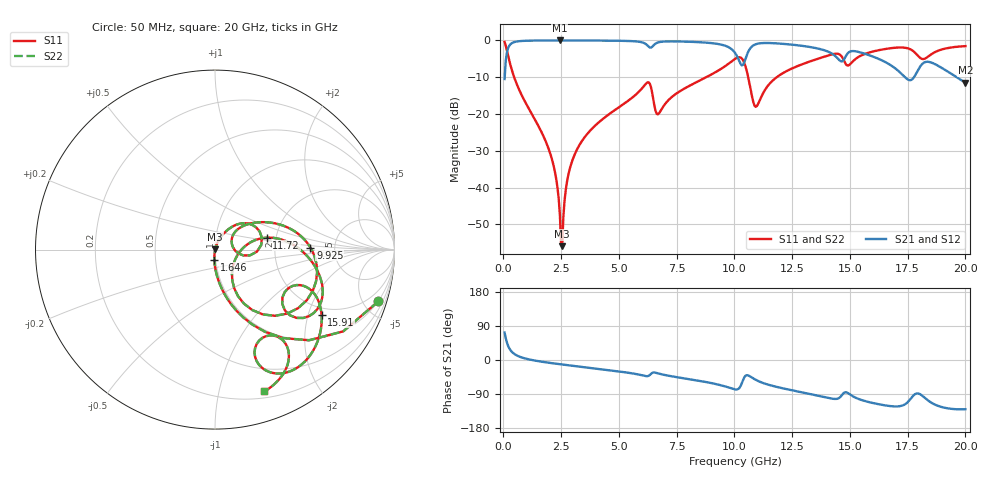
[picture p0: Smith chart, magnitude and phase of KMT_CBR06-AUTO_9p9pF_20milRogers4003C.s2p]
! Data measured by Modelithics Inc. support@modelithics.com 813-866-6335
! KEMET CBR06-AUTO 9.9pF, Pad Width= 0.851mm, Pad Length= 0.64mm, Pad Gap= 0.62mm, 20mil Rogers 4003C substrate Data, January 2022
# hz S ma R 50
! 2 Port Network Data from SP1.SP block
! freq  magS11  angS11  magS21  angS21  magS12  angS12  magS22  angS22
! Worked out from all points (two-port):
!   401 points, 50 MHz to 20 GHz, reference 50 ohm
!   highest |S21| = -0.01 dB at 2.444 GHz (marker M1); lowest = -11.5 dB at 20 GHz (marker M2)
!   |S21| within 3 dB of the highest: 161.7 MHz to 9.978 GHz (9.817 GHz wide, 194 % of centre); 10.6 GHz to 14.04 GHz (3.435 GHz wide, 27.9 % of centre)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
!   lowest |S11| = -55.9 dB at 2.544 GHz (marker M3), VSWR 1.00, Z = 50.1 + j0.102 ohm
!   |S11| at or under -10 dB: 463.8 MHz to 8.779 GHz (8.315 GHz wide, 180 % of centre); 10.6 GHz to 11.83 GHz (1.237 GHz wide, 11 % of centre)
!   |S22| runs from -55.9 to -0.4 dB; largest |S21 - S12| = 0
!   S11 on the Smith chart (normalised r, x): 50 MHz: 0.98, -6.30; 1.646 GHz: 0.99, -0.11; 9.925 GHz: 3.27, +0.10; 11.72 GHz: 1.79, +0.26; 15.91 GHz: 1.75, -2.45; 20 GHz: 0.26, -1.37
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5e7  0.9542 -17.6  0.2989 72.4  0.2989 72.4  0.9542 -17.6
4.49e8  0.3259 -73.0  0.9448 16.9  0.9448 16.9  0.3259 -73.0
1.646e9  0.05689 -93.6  0.9975 -4.4  0.9975 -4.4  0.05689 -93.6
2.194625e9  0.01839 -96.3  0.9988 -9.1  0.9988 -9.1  0.01839 -96.3
2.444e9  0.004223 -87.8  0.9989 -11.1  0.9989 -11.1  0.004223 -87.8
2.54375e9  0.001595 39.7  0.9989 -11.9  0.9989 -11.9  0.001595 39.7
2.843e9  0.01653 72.2  0.9987 -14.1  0.9987 -14.1  0.01653 72.2
3.391625e9  0.04259 70.2  0.9978 -18.2  0.9978 -18.2  0.04259 70.2
6.2345e9  0.2686 21.8  0.8543 -42.7  0.8543 -42.7  0.2686 21.8
6.73325e9  0.102 24.7  0.9459 -36.0  0.9459 -36.0  0.102 24.7
9.92525e9  0.5317 1.2  0.7372 -76.0  0.7372 -76.0  0.5317 1.2
1.0025e10  0.5601 -4.9  0.677 -77.5  0.677 -77.5  0.5601 -4.9
1.0424e10  0.498 -47.8  0.5017 -46.0  0.5017 -46.0  0.498 -47.8
1.092275e10  0.1251 -24.9  0.8869 -52.3  0.8869 -52.3  0.1251 -24.9
1.172075e10  0.2965 13.0  0.9159 -69.4  0.9159 -69.4  0.2965 13.0
1.336662e10  0.5305 -5.7  0.804 -90.9  0.804 -90.9  0.5305 -5.7
1.486288e10  0.4603 -35.3  0.6408 -85.6  0.6408 -85.6  0.4603 -35.3
1.591025e10  0.6952 -31.3  0.6171 -112.3  0.6171 -112.3  0.6952 -31.3
1.670825e10  0.7795 -44.5  0.4729 -121.4  0.4729 -121.4  0.7795 -44.5
1.790525e10  0.6382 -69.5  0.3737 -88.2  0.3737 -88.2  0.6382 -69.5
1.845388e10  0.6248 -53.3  0.508 -109.8  0.508 -109.8  0.6248 -53.3
2e10  0.8367 -70.8  0.2651 -129.8  0.2651 -129.8  0.8367 -70.8
